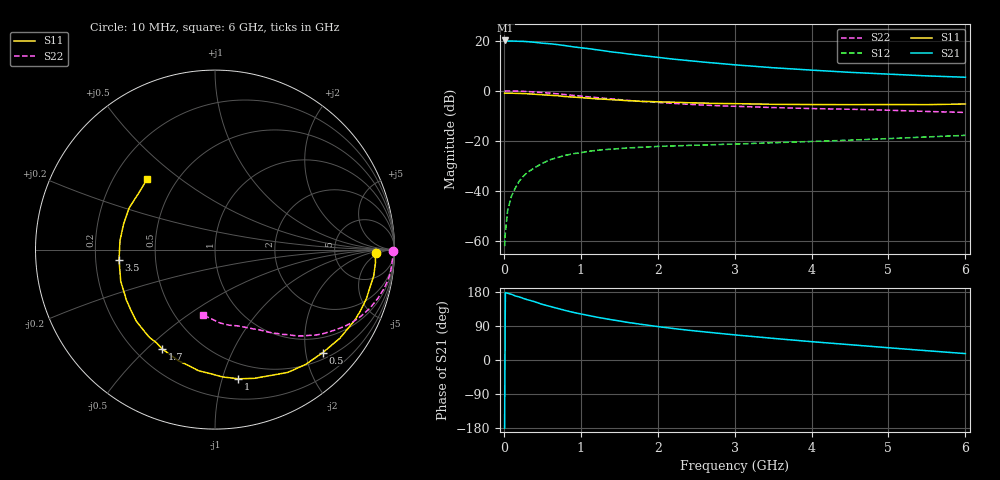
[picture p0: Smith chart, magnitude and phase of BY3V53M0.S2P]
! SIEMENS Small Signal Semiconductors
! BFY420
! Si NPN RF SIEGET Grounded Emitter Transistor in MICRO-X
! VCE = 3.5 V  IC = 3 mA
! Common Emitter S-Parameters:  October  1996
# GHz  S  MA  R  50
!  f  S11  S21  S12  S22
! GHz  MAG  ANG  MAG  ANG  MAG  ANG  MAG  ANG
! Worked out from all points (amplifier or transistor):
!   36 points, 10 MHz to 6 GHz, reference 50 ohm
!   highest |S21| = 20.1 dB at 20 MHz (marker M1)
!   |S21| within 3 dB of that: start of sweep to 1.028 GHz
!   unconditionally stable (mu >= 1): 3.634 GHz to end of sweep
!   at 250 MHz: K = 0.09, MSG = 26.9 dB, |S12| = -34.2 dB
!   at 1.4 GHz: K = 0.38, MSG = 19.4 dB, |S12| = -23.3 dB
!   at 6 GHz: K = 1.18, MAG = 9.0 dB, |S12| = -17.8 dB
!   S11 on the Smith chart (normalised r, x): 10 MHz: 18, -3; 500 MHz: 0.63, -2.35; 1 GHz: 0.36, -1.13; 1.7 GHz: 0.31, -0.56; 3.5 GHz: 0.30, -0.05; 6 GHz: 0.34, +0.38
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0.01  0.8958 -1.1  10.06 -180.0  0.0008 72.9  0.9925 -0.4
0.02  0.8934 -2.1  10.07 178.1  0.0015 77.5  0.9859 -0.8
0.05  0.8971 -4.6  9.81 175.9  0.0042 83.7  0.9925 -2.1
0.1  0.8964 -9.4  9.818 173.4  0.008 82.5  0.9886 -4.4
0.15  0.8886 -13.6  9.744 168.9  0.0116 79.7  0.9866 -6.6
0.2  0.8867 -17.9  9.677 166.5  0.0158 79.2  0.9824 -8.6
0.3  0.8725 -26.8  9.541 159.5  0.0232 74.9  0.9672 -12.9
0.4  0.8534 -35.3  9.252 153.8  0.0293 71.0  0.9458 -16.9
0.5  0.8308 -43.7  8.891 146.8  0.0358 65.8  0.9226 -20.7
0.7  0.7956 -59.3  8.324 136.1  0.0469 59.0  0.8684 -27.6
0.8  0.766 -66.4  7.928 130.7  0.0516 54.8  0.8397 -30.6
1  0.7317 -79.7  7.205 121.6  0.0582 49.3  0.7837 -35.8
1.1  0.7107 -86.6  6.923 117.5  0.0622 46.6  0.7586 -38.3
1.4  0.6627 -102.9  5.952 106.2  0.0684 40.4  0.6895 -44.2
1.7  0.6272 -117.8  5.239 96.7  0.0737 36.3  0.6276 -49.1
2  0.6022 -130.6  4.64 88.2  0.0778 32.7  0.5843 -53.2
2.2  0.5926 -137.7  4.276 83.2  0.0796 31.1  0.5615 -55.7
2.8  0.5579 -156.1  3.507 70.3  0.085 28.4  0.5019 -62.2
3.5  0.5376 -174.1  2.879 57.1  0.0921 26.6  0.4628 -69.0
4.5  0.5289 164.1  2.331 40.4  0.1038 24.5  0.4286 -79.4
5.5  0.5293 143.2  1.98 24.5  0.1201 22.2  0.3871 -92.6
6  0.5452 133.9  1.86 16.9  0.1294 20.3  0.37 -100.4
